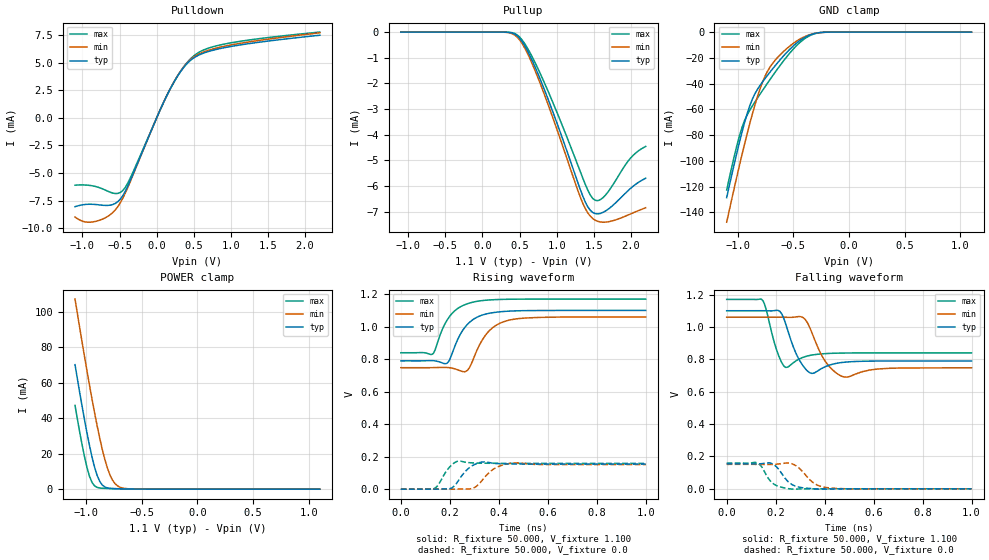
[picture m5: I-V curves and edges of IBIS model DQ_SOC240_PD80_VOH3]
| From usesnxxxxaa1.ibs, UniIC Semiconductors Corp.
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|   Model DQ_SOC240_PD80_VOH3
[Model] DQ_SOC240_PD80_VOH3
Model_type I/O
Polarity   Non-Inverting
Enable   Active-High
Vinl =  0.113V
Vinh =  0.253V
Vmeas =  0.183V
Rref =  50.000
Vref =  0.183V
C_comp   1.110pF   1.087pF   1.118pF
[Model Spec]
Vinh   0.253V   0.247V   0.265V
Vinl   0.113V   0.107V   0.125V
Vmeas   0.183V   NA   NA
Vref   0.183V   NA   NA
Rref   50.000   NA   NA
[Temperature Range]   25.000   0.125k   -40.000
[Voltage Range]   1.100V   1.060V   1.170V
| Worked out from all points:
|   slope of the pulldown table from 0 to 0.165 V, typ, clamps not added: 68.6 ohm
|   GND clamp passes 1 mA (typ) near -0.30 V on its own axis
|   POWER clamp passes 1 mA (typ) near -0.82 V on its own axis
|   rising waveform, R_fixture 50.000, V_fixture 1.100: 20-80 % time 76.2ps typ, 79.9ps min, 74.5ps max; typ from 0.79 V to 1.1 V
|   rising waveform, R_fixture 50.000, V_fixture 0.0: 20-80 % time 48.1ps typ, 58.4ps min, 38.9ps max; typ from 0 V to 0.154 V
|   falling waveform, R_fixture 50.000, V_fixture 1.100: 20-80 % time 42.2ps typ, 54.8ps min, 32.3ps max; typ from 1.1 V to 0.79 V
|   falling waveform, R_fixture 50.000, V_fixture 0.0: 20-80 % time 51.3ps typ, 60.3ps min, 43.6ps max; typ from 0.154 V to 0 V
[Pulldown]
|Voltage   I(typ)   I(min)   I(max)
-1.1V     -8.06mA    -9.005mA   -6.106mA
-930mV    -7.843mA   -9.47mA    -6.107mA
-726mV    -7.932mA   -9.181mA   -6.449mA
-556mV    -7.761mA   -8.341mA   -6.868mA
-454mV    -7.04mA    -7.266mA   -6.58mA
-352mV    -5.637mA   -5.732mA   -5.417mA
158mV     2.314mA    2.324mA    2.293mA
328mV     4.261mA    4.301mA    4.293mA
498mV     5.443mA    5.524mA    5.628mA
668mV     5.978mA    6.084mA    6.272mA
940mV     6.421mA    6.553mA    6.75mA
2.2V      7.518mA    7.735mA    7.803mA
[Pullup]
|Voltage   I(typ)   I(min)   I(max)
-1.1V     -58.82pA   10.24nA    0A
432mV     -74.32uA   -110.7uA   -50.31uA
568mV     -523.4uA   -612.1uA   -444.4uA
738mV     -1.552mA   -1.706mA   -1.362mA
976mV     -3.321mA   -3.56mA    -2.93mA
1.316V    -6.107mA   -6.406mA   -5.413mA
1.418V    -6.797mA   -7.033mA   -6.143mA
1.486V    -7.024mA   -7.26mA    -6.478mA
1.554V    -7.079mA   -7.37mA    -6.564mA
1.622V    -7.025mA   -7.403mA   -6.455mA
1.996V    -6.088mA   -7.082mA   -4.908mA
2.2V      -5.692mA   -6.84mA    -4.454mA
[GND_clamp]
|Voltage   I(typ)   I(min)   I(max)
-1.1V     -128.5mA   -147.6mA   -122.6mA
-1.008V   -93.62mA   -112mA     -87.95mA
-962mV    -77.6mA    -95.05mA   -73.96mA
-893mV    -57.36mA   -71.21mA   -60.7mA
-847mV    -48.01mA   -56.81mA   -54.36mA
-801mV    -41.47mA   -44.23mA   -48.33mA
-755mV    -36.02mA   -34.19mA   -42.41mA
-709mV    -30.9mA    -26.94mA   -36.63mA
-525mV    -12.67mA   -10.3mA    -15.49mA
-387mV    -3.615mA   -3.065mA   -4.419mA
-249mV    -281uA     -330.6uA   -301.3uA
1.1V      0A         0A         0A
[POWER_clamp]
|Voltage   I(typ)   I(min)   I(max)
-1.1V     70.27mA    107.3mA    47.25mA
-1.039V   47.68mA    83.93mA    25.86mA
-993mV    31.88mA    66.94mA    12.35mA
-970mV    24.65mA    58.72mA    7.262mA
-947mV    18.06mA    50.74mA    3.761mA
-901mV    7.73mA     35.71mA    987.1uA
-855mV    2.348mA    22.46mA    514uA
-809mV    697.3uA    11.94mA    396.5uA
-763mV    321uA      5.097mA    322.7uA
-717mV    213.8uA    1.813mA    258.1uA
-556mV    65.24uA    79.15uA    81.64uA
1.1V      0A         0A         0A
[Ramp]
| variable   typ   min   max
dV/dt_r   92.531m/48.180p   90.527m/58.643p   95.291m/38.949p
dV/dt_f   0.186/42.420p   0.187/54.879p   0.198/32.547p
R_load = 50.000
[Rising Waveform]
R_fixture= 50.000
V_fixture= 1.100
V_fixture_min= 1.060
V_fixture_max= 1.170
|time   V(typ)   V(min)   V(max)
0s        789.7mV    747.6mV    839.6mV
130ps     791mV      747.9mV    831.7mV
189ps     775.2mV    748.8mV    1.041V
262ps     996.6mV    722.7mV    1.136V
281ps     1.027V     750mV      1.146V
300ps     1.049V     816mV      1.153V
331ps     1.071V     914.4mV    1.16V
366ps     1.084V     982.1mV    1.165V
447ps     1.096V     1.042V     1.169V
1ns       1.1V       1.06V      1.17V
[Rising Waveform]
R_fixture= 50.000
V_fixture= 0.0
V_fixture_min= 0.0
V_fixture_max= 0.0
|time   V(typ)   V(min)   V(max)
0s        2.545uV    20.59uV    475.2nV
138ps     117.3uV    -14.03uV   5.044mV
201ps     3.326mV    147.3uV    139mV
235ps     52.2mV     624.1uV    172.7mV
275ps     126.3mV    1.205mV    163.6mV
302ps     152.4mV    10.86mV    161.1mV
322ps     163.8mV    36.58mV    160.2mV
378ps     159.6mV    122.8mV    159.2mV
448ps     154.8mV    159.1mV    158.9mV
1ns       154.2mV    150.9mV    158.8mV
[Falling Waveform]
R_fixture= 50.000
V_fixture= 1.100
V_fixture_min= 1.060
V_fixture_max= 1.170
|time   V(typ)   V(min)   V(max)
0s        1.1V       1.06V      1.17V
148ps     1.1V       1.06V      1.162V
217ps     1.097V     1.06V      805.5mV
241ps     1.019V     1.06V      749.6mV
293ps     805.9mV    1.064V     799.3mV
349ps     712.7mV    960.7mV    826.4mV
407ps     757.1mV    778.5mV    835.5mV
478ps     781.6mV    691.3mV    838.6mV
615ps     789.1mV    739.8mV    839.6mV
1ns       789.7mV    747.5mV    839.6mV
[Falling Waveform]
R_fixture= 50.000
V_fixture= 0.0
V_fixture_min= 0.0
V_fixture_max= 0.0
|time   V(typ)   V(min)   V(max)
0s        154.2mV    150.9mV    158.8mV
123ps     153.7mV    150.8mV    161.3mV
144ps     155.6mV    150.5mV    133.7mV
183ps     157.1mV    150.5mV    41.16mV
211ps     123.2mV    153.3mV    15.23mV
258ps     35mV       157.9mV    -355uV
292ps     11.58mV    132.6mV    -1.228mV
359ps     -408uV     31.88mV    -156.3uV
399ps     -2.136mV   9.471mV    -44.93uV
1ns       2.705uV    21.33uV    802.9nV
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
